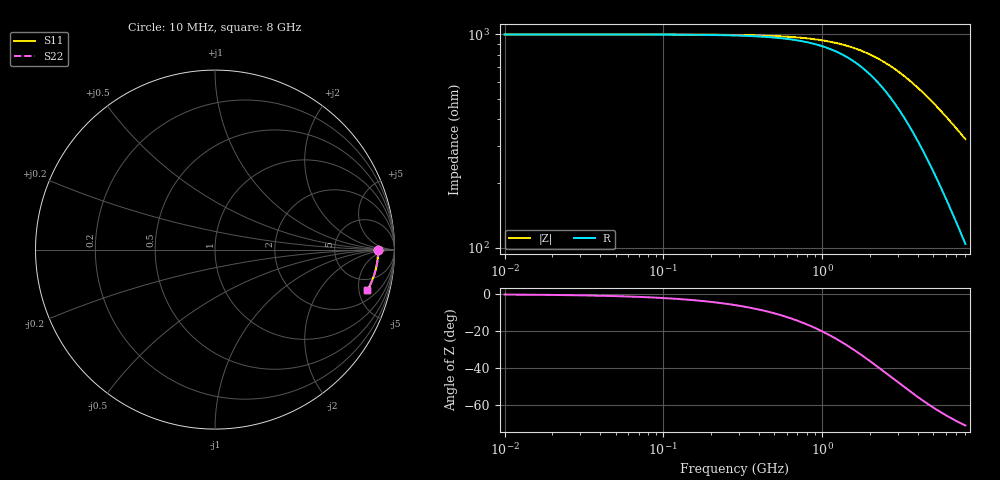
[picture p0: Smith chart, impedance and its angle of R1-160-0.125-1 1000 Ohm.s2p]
!version-1
!date-03.2021
# MHz S RI R 50
!Freq ReS11 ImS11 ReS21 ImS21 ReS12 ImS12 ReS22 ImS22
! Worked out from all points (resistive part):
!   800 points, 10 MHz to 8 GHz, reference 50 ohm
!   read as one part in series: R = 1 kohm at 50 MHz
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10  0.9091 -0.000305  0.0909 0.000303  0.0909 0.000303  0.9091 -0.000303
160  0.9091 -0.00488  0.0909 0.00484  0.0909 0.00484  0.9091 -0.00485
320  0.909 -0.00975  0.091 0.00969  0.091 0.00969  0.909 -0.00969
480  0.9089 -0.0146  0.0911 0.0145  0.0911 0.0145  0.9089 -0.0145
640  0.9087 -0.0195  0.0913 0.0194  0.0913 0.0194  0.9087 -0.0194
810  0.9084 -0.0247  0.0916 0.0245  0.0916 0.0245  0.9084 -0.0245
980  0.9081 -0.0298  0.0919 0.0296  0.0919 0.0296  0.9081 -0.0297
1160  0.9077 -0.0353  0.0923 0.0351  0.0923 0.0351  0.9077 -0.0351
1350  0.9072 -0.0411  0.0927 0.0408  0.0927 0.0408  0.9073 -0.0408
1600  0.9065 -0.0486  0.0935 0.0483  0.0935 0.0483  0.9065 -0.0483
1890  0.9055 -0.0574  0.0945 0.057  0.0945 0.057  0.9055 -0.057
2210  0.9042 -0.067  0.0958 0.0665  0.0958 0.0665  0.9042 -0.0666
2680  0.9019 -0.081  0.0981 0.0805  0.0981 0.0805  0.9019 -0.0805
3420  0.8974 -0.1029  0.1026 0.1022  0.1026 0.1022  0.8975 -0.1023
4010  0.8931 -0.1201  0.1069 0.1193  0.1069 0.1193  0.8932 -0.1193
4680  0.8874 -0.1393  0.1125 0.1383  0.1125 0.1383  0.8876 -0.1384
5340  0.8811 -0.1578  0.1188 0.1567  0.1188 0.1567  0.8812 -0.1568
6000  0.874 -0.1759  0.1259 0.1747  0.1259 0.1747  0.8742 -0.1748
6670  0.8661 -0.1938  0.1338 0.1924  0.1338 0.1924  0.8664 -0.1925
7390  0.8569 -0.2124  0.1429 0.2109  0.1429 0.2109  0.8572 -0.2111
7840  0.8508 -0.2237  0.1491 0.2222  0.1491 0.2222  0.8511 -0.2223
8000  0.8485 -0.2277  0.1513 0.2261  0.1513 0.2261  0.8489 -0.2263
